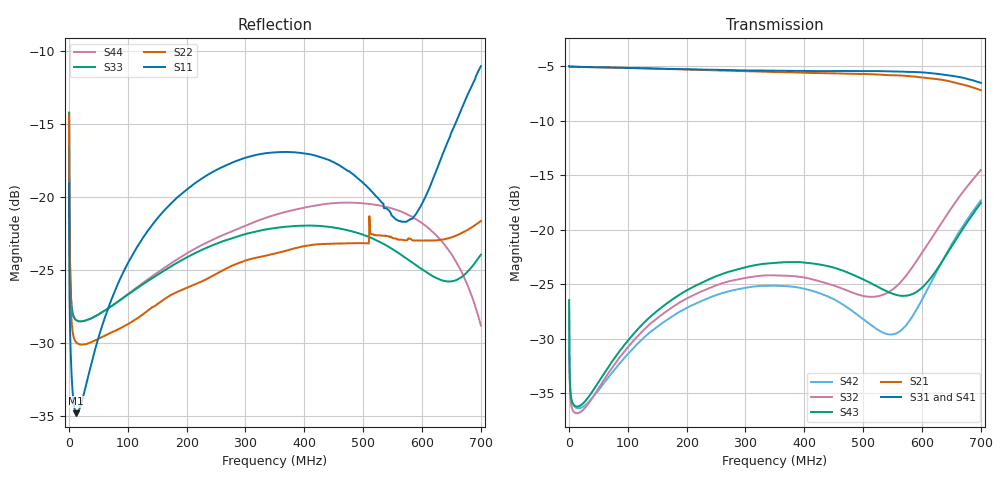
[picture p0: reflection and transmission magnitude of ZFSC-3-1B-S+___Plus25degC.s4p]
!MINI-CIRCUITS
!MODEL: ZFSC-3-1B-S+, RUN#F08810
!PORT-1=S , PORT-2=1, PORT-3=2,PORT-4=3
!Agilent Technologies,N5230A,MY45001447,A.07.50.63
!Agilent N5230A: A.07.50.63
!Date: Tuesday, February 08, 2011 11:58:04
!Correction: S11(Full 4 Port(1,2,3,4))
!S12(Full 4 Port(1,2,3,4))
!S13(Full 4 Port(1,2,3,4))
!S14(Full 4 Port(1,2,3,4))
!S21(Full 4 Port(1,2,3,4))
!S22(Full 4 Port(1,2,3,4))
!S23(Full 4 Port(1,2,3,4))
!S24(Full 4 Port(1,2,3,4))
!S31(Full 4 Port(1,2,3,4))
!S32(Full 4 Port(1,2,3,4))
!S33(Full 4 Port(1,2,3,4))
!S34(Full 4 Port(1,2,3,4))
!S41(Full 4 Port(1,2,3,4))
!S42(Full 4 Port(1,2,3,4))
!S43(Full 4 Port(1,2,3,4))
!S44(Full 4 Port(1,2,3,4))
!S4P File: Measurements: <S11,S12,S13,S14>,
!<S21,S22,S23,S24>,
!<S31,S32,S33,S34>,
!<S41,S42,S43,S44>:
# Hz S  dB  R 50
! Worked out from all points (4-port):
!   1406 points, 300 kHz to 700 MHz, reference 50 ohm
!   strongest paths, dB at 300 kHz, 173 MHz, 349 MHz, 524.5 MHz, 700 MHz:
!     S31: -5.0, -5.2, -5.4, -5.4, -6.5
!     S41: -5.0, -5.2, -5.5, -5.6, -6.9
!     S21: -5.0, -5.2, -5.5, -5.8, -7.2
!     S43: -26.5, -26.5, -23.1, -25.2, -17.5
!     S32: -27.3, -27.2, -24.2, -26.1, -14.5
!     S42: -27.3, -28.1, -25.2, -29.2, -17.3
!   lowest |S11| = -34.8 dB at 12.5 MHz (marker M1), VSWR 1.04, Z = 49.2 + j1.64 ohm
!   |S11| at or under -10 dB: start of sweep to end of sweep
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300000  -19.05 105.8  -4.96 6.1  -4.96 6.1  -4.96 6.1
        -4.99 6.2  -14.33 110.4  -27.29 -56.2  -27.23 -56.9
        -4.99 6.3  -27.27 -56.4  -14.25 109.4  -26.40 -56.3
        -4.99 6.2  -27.31 -57.1  -26.47 -56.2  -14.21 109.4
4500000  -32.16 125.8  -5.02 -0.6  -5.02 -0.6  -5.02 -0.6
         -5.02 -0.6  -28.51 49.7  -36.32 -163.3  -35.71 -163.9
         -5.02 -0.6  -36.34 -163.3  -27.47 44.6  -35.63 -162.6
         -5.01 -0.6  -35.74 -164.1  -35.65 -162.7  -27.42 44.3
1.25e7  -34.80 113.9  -5.04 -2.5  -5.04 -2.7  -5.04 -2.6
        -5.04 -2.5  -29.95 21.1  -36.85 169.8  -36.35 170.9
        -5.04 -2.7  -36.86 169.5  -28.44 19.6  -36.24 169.5
        -5.04 -2.6  -36.38 170.7  -36.25 169.4  -28.43 19.4
1.63e8  -20.88 50.6  -5.23 -32.5  -5.22 -33.7  -5.23 -33.0
        -5.24 -32.5  -26.96 1.9  -27.59 80.3  -28.39 80.4
        -5.22 -33.7  -27.60 80.3  -25.01 10.8  -26.89 77.6
        -5.24 -33.0  -28.42 80.3  -26.91 77.7  -24.82 10.7
4.155e8  -17.13 -22.7  -5.59 -85.1  -5.43 -87.3  -5.52 -85.0
         -5.61 -85.0  -23.27 -55.0  -24.59 40.4  -25.65 30.6
         -5.43 -87.3  -24.59 40.3  -21.96 -38.3  -23.10 29.0
         -5.53 -84.9  -25.66 30.6  -23.12 29.1  -20.60 -35.1
5.58e8  -21.59 -111.3  -5.84 -122.2  -5.47 -123.9  -5.67 -119.7
        -5.83 -122.2  -22.89 -118.5  -25.12 73.2  -29.46 60.3
        -5.47 -124.2  -25.14 73.0  -23.78 -94.6  -26.02 36.9
        -5.65 -119.8  -29.48 60.1  -26.02 37.0  -20.90 -75.1
7e8  -11.05 108.1  -7.22 -173.4  -6.51 -173.0  -6.88 -165.1
     -7.19 -173.8  -21.64 134.3  -14.47 78.1  -17.28 80.6
     -6.52 -173.5  -14.52 78.0  -23.95 133.2  -17.54 69.0
     -6.87 -165.5  -17.32 80.5  -17.53 69.1  -28.80 -133.9
